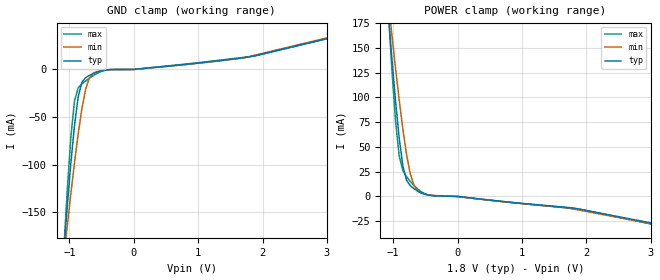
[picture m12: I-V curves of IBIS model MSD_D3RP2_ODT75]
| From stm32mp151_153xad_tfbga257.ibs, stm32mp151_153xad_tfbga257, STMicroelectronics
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[Model] MSD_D3RP2_ODT75
Model_type   Input
C_comp 2.151pF   2.088pF   2.212pF
Vinh = 1.150V
Vinl = 650.000mV
[Model Spec]
Vinh   1.150V   1.100V   1.200V
Vinl   650.000mV   600.000mV   700.000mV
[Temperature Range]   25.000   125.000   -40.000
[Voltage Range]   1.800V   1.700V   1.900V
[GND Clamp Reference]   0.00V   0.00V   0.00V
[POWER Clamp Reference]   1.800V   1.700V   1.900V
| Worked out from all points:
|   GND clamp passes 1 mA (typ) near -0.47 V on its own axis
|   POWER clamp passes 1 mA (typ) near -0.41 V on its own axis
[GND Clamp]
-1.785V   -869.9mA   -658.6mA   -1.174A
-1.094V   -197mA     -202.2mA   -198mA
-1.036V   -146.4mA   -166.3mA   -130mA
-978.8mV  -99.48mA   -131.4mA   -72.26mA
-921.2mV  -59.06mA   -98.19mA   -33.11mA
-863.6mV  -28.89mA   -67.64mA   -19.32mA
-806.1mV  -13.55mA   -41.19mA   -15.17mA
-748.5mV  -8.607mA   -21.01mA   -12.11mA
-690.9mV  -6.288mA   -9.088mA   -9.265mA
-460.6mV  -815.7uA   -658.5uA   -1.147mA
1.785V    13.01mA    13.44mA    13.36mA
3.57V     41.37mA    42.41mA    41.62mA
[Power Clamp]
-1.77V    836.6mA    647.1mA    1.106A
-1.079V   188mA      199.5mA    191.8mA
-1.021V   140.5mA    164.2mA    129.7mA
-963.6mV  96.89mA    130mA      76.58mA
-906.1mV  58.97mA    97.41mA    40.92mA
-848.5mV  30.58mA    67.58mA    26.09mA
-790.9mV  16.27mA    41.99mA    19.93mA
-733.3mV  10.9mA     22.68mA    15.17mA
-618.2mV  5.355mA    5.744mA    7.475mA
-387.9mV  869.8uA    1.034mA    821uA
1.8V      -11.65mA   -12.68mA   -12.23mA
3.585V    -34.03mA   -34.7mA    -35.72mA
